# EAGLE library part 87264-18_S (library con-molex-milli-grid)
RECEPTACAL
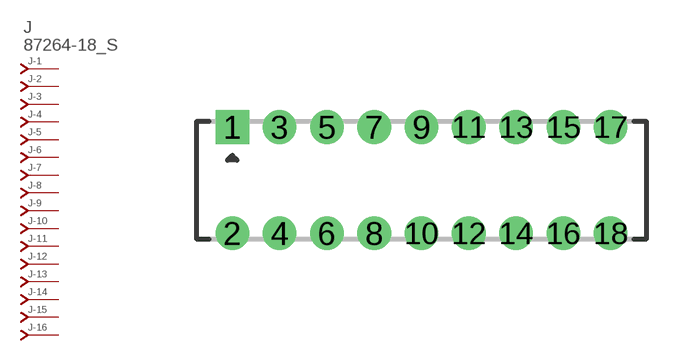
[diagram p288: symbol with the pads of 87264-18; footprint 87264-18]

Designator prefix J; gates -1=J-NV -2=J-N -3=J-N -4=J-N -5=J-N -6=J-N -7=J-N -8=J-N -9=J-N -10=J-N -11=J-N -12=J-N -13=J-N -14=J-N -15=J-N -16=J-N -17=J-N -18=J-N

## 87264-18_S  [87264-18]
1  -1:J  pas
2  -2:J  pas
3  -3:J  pas
4  -4:J  pas
5  -5:J  pas
6  -6:J  pas
7  -7:J  pas
8  -8:J  pas
9  -9:J  pas
10  -10:J  pas
11  -11:J  pas
12  -12:J  pas
13  -13:J  pas
14  -14:J  pas
15  -15:J  pas
16  -16:J  pas
17  -17:J  pas
18  -18:J  pas

## Footprint 87264-18 (pad centres in mm)
RECEPTACAL Dual Row, Side Entry
drill 0.914 square: 1 -8,2.25
drill 0.914: 2 -8,-2.25; 3 -6,2.25; 4 -6,-2.25; 5 -4,2.25; 6 -4,-2.25; 7 -2,2.25; 8 -2,-2.25; 9 0,2.25; 10 0,-2.25; 11 2,2.25; 12 2,-2.25; 13 4,2.25; 14 4,-2.25; 15 6,2.25; 16 6,-2.25; 17 8,2.25; 18 8,-2.25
